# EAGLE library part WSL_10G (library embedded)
Connector WSL 10G WANNENSTECKER, 10-POLIG BOX HEADER Source: Box Header
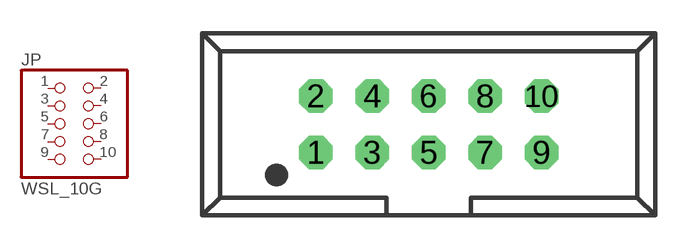
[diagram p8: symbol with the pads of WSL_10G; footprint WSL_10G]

Designator prefix JP

## WSL_10G (ANGLE: Straight; DATASHEET: https://cdn-reichelt.de/documents/datenblatt/C151/BH1S-XX-L.pdf; DESCR: Box connector 10pin straight; MF: Amtek; MF_PN: WSL-10G; PACKAGE: Box Header; PITCH: 2.54mm; POS: 10; PURCHASE: https://www.reichelt.de/box-connector-10-pin-straight-wsl-10g-p22816.html?r=1; REICHELT_NO: WSL 10G; ROWS: 2; UNIT_PRICE: 0.1)  [WSL_10G]
1  1  pas
2  2  pas
3  3  pas
4  4  pas
5  5  pas
6  6  pas
7  7  pas
8  8  pas
9  9  pas
10  10  pas

## Footprint WSL_10G (pad centres in mm)
CONNECTOR series 057 contact pc board low profile headers straight
drill 1 octagon: 1 -5.08,-1.27; 2 -5.08,1.27; 3 -2.54,-1.27; 4 -2.54,1.27; 5 0,-1.27; 6 0,1.27; 7 2.54,-1.27; 8 2.54,1.27; 9 5.08,-1.27; 10 5.08,1.27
